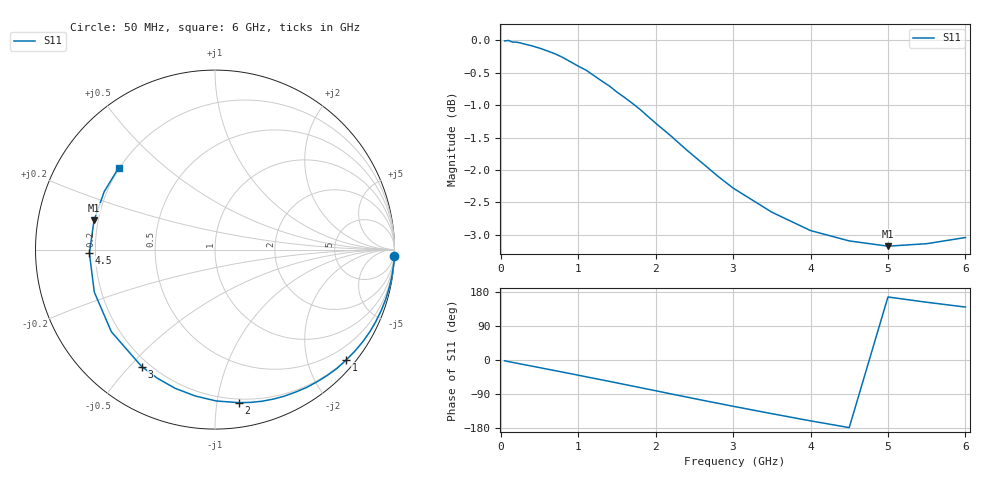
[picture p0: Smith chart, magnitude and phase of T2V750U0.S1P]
! SIEMENS Discrete & RF Semiconductors
! BAS70-04W
! Si Schottky Diode in SOT323
! VR = 0.75 V
! S-Parameters:  November  1997
# GHz  S  MA  R  50
!  f  S11
! GHz  MAG  ANG
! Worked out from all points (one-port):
!   34 points, 50 MHz to 6 GHz, reference 50 ohm
!   lowest |S11| = -3.2 dB at 5 GHz (marker M1), VSWR 5.53, Z = 9.17 + j5.81 ohm
!   |S11| at or under -10 dB: nowhere
!   S11 on the Smith chart (normalised r, x): 50 MHz: 1, -55; 1 GHz: 0.19, -2.73; 2 GHz: 0.17, -1.15; 3 GHz: 0.17, -0.54; 4.5 GHz: 0.18, -0.01; 6 GHz: 0.20, +0.35
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0.05  0.9991 -2.1
0.1  1 -4.1
0.2  0.9969 -8.1
0.3  0.9938 -12.1
0.4  0.9905 -16.1
0.5  0.9864 -20.0
0.6  0.9817 -24.1
0.7  0.9766 -28.0
0.8  0.9702 -32.0
1  0.9554 -40.1
1.1  0.9486 -44.2
1.3  0.9307 -52.2
1.4  0.9224 -56.3
1.6  0.9034 -64.6
1.7  0.8941 -68.7
1.8  0.8844 -72.8
2  0.8632 -81.1
2.2  0.8435 -89.5
2.4  0.823 -97.7
2.6  0.8042 -106.0
2.8  0.7857 -114.0
3  0.7691 -122.1
3.5  0.7368 -141.6
4  0.713 -160.6
4.5  0.7 -178.4
5  0.6935 166.3
5.5  0.6966 152.4
6  0.7043 139.7
